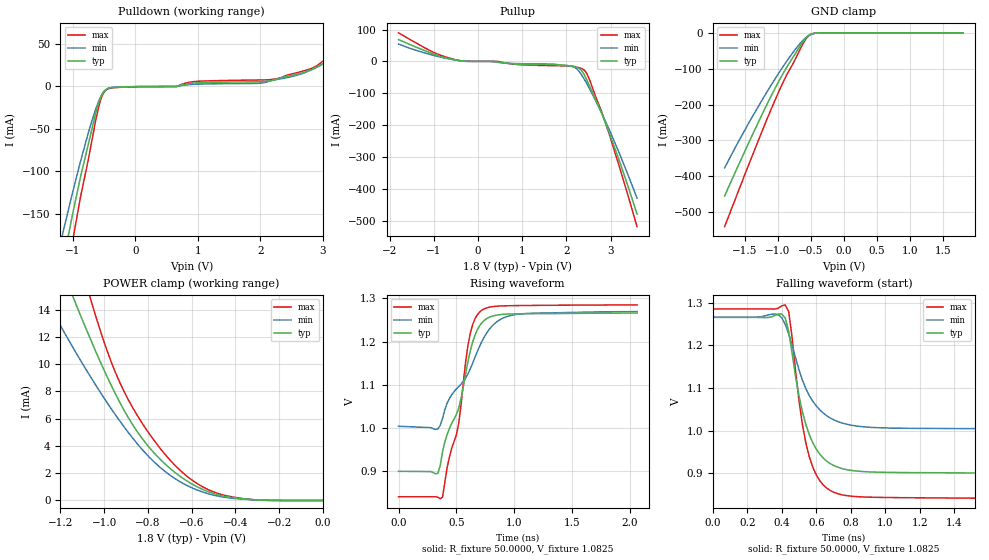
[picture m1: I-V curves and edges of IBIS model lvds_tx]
| Texas Instruments Incorporated
| 10bit, w200-MSPS, 4-channel/ 12bit, 80-MSPS, 8-Channel ADC
| Marketing part#   Voltage Range   Package-type   #pins/pkg drawing
| ADS5296   1.7V - 1.9V   QFN   64/QFN
[IBIS ver] 4.1
[File name] ads5296.ibs
[File Rev] 1.0
[Date] Mon Nov 16 17:09:14 IST 2009
[Source]   TIspice3 simulations
   Texas Instruments Incorporated.
   Analog eLab Design Center, HPA
   12500 TI Blvd
   Dallas, TX -75243
   For Support e-mail: elab_scm_ibis@list.ti.com
[Disclaimer]  Please be aware that in the absence of a written agreement,
   Texas Instruments (TI) assumes no liability for: 1)
   the accuracy of the IBIS models provided to your company, 2)
   the proper functioning of these IBIS models in your design or
   for any resulting applications, or; 3) infringement of patents,
   copyrights, or intellectual property rights resulting from
   your use of these IBIS models. TI provides IBIS models as a
   service to our customers and therefore reserves the right to
   limit distribution of the IBIS models.
[Copyright] (C)Copyright 2013 Texas Instruments Incorporated.
   All rights reserved.
|   Component ADS529xIPFP
[Component] ADS529xIPFP
[Manufacturer] Texas Instruments.
[Package]
| variable   typ   min   max
R_pkg   0.3702   0.1484   0.5035
L_pkg   3.6148nH   2.8818nH   4.60713nH
C_pkg   0.6034pF   0.5489pF   0.7199pF
[Pin]  signal_name   model_name   R_pin   L_pin   C_pin
1   TERM   TERM   NA   NA   NA
2   TERM   TERM   NA   NA   NA
3   TERM   TERM   NA   NA   NA
4   TERM   TERM   NA   NA   NA
5   TERM   TERM   NA   NA   NA
6   AGND   GND   NA   NA   NA
7   TERM   TERM   NA   NA   NA
8   TERM   TERM   NA   NA   NA
9   AGND   GND   NA   NA   NA
10   TERM   TERM   NA   NA   NA
11   TERM   TERM   NA   NA   NA
12   LGND   GND   NA   NA   NA
13   TERM   TERM   NA   NA   NA
14   LGND   GND   NA   NA   NA
15   OUT0_P   lvds_tx   NA   NA   NA
16   OUT0_N   lvds_tx   NA   NA   NA
17   OUT1_P   lvds_tx   NA   NA   NA
18   OUT1_N   lvds_tx   NA   NA   NA
19   OUT2_P   lvds_tx   NA   NA   NA
20   OUT2_N   lvds_tx   NA   NA   NA
21   OUT3_P   lvds_tx   NA   NA   NA
22   OUT3_N   lvds_tx   NA   NA   NA
23   ADCLKP   lvds_tx   NA   NA   NA
24   ADCLKN   lvds_tx   NA   NA   NA
25   LCLKP   lvds_tx   NA   NA   NA
26   LCLKN   lvds_tx   NA   NA   NA
27   OUT4_P   lvds_tx   NA   NA   NA
28   OUT4_N   lvds_tx   NA   NA   NA
29   OUT5_P   lvds_tx   NA   NA   NA
30   OUT5_N   lvds_tx   NA   NA   NA
31   OUT6_P   lvds_tx   NA   NA   NA
32   OUT6_N   lvds_tx   NA   NA   NA
33   OUT7_P   lvds_tx   NA   NA   NA
34   OUT7_N   lvds_tx   NA   NA   NA
35   LVDD   POWER   NA   NA   NA
36   LGND   GND   NA   NA   NA
37   AGND   GND   NA   NA   NA
38   TERM   TERM   NA   NA   NA
39   TERM   TERM   NA   NA   NA
40   AGND   GND   NA   NA   NA
41   TERM   TERM   NA   NA   NA
42   TERM   TERM   NA   NA   NA
43   AGND   GND   NA   NA   NA
44   TERM   TERM   NA   NA   NA
45   TERM   TERM   NA   NA   NA
46   AGND   GND   NA   NA   NA
47   TERM   TERM   NA   NA   NA
48   TERM   TERM   NA   NA   NA
49   TERM   TERM   NA   NA   NA
50   AVDD   POWER   NA   NA   NA
51   NC   NC   NA   NA   NA
52   TERM   TERM   NA   NA   NA
53   TERM   TERM   NA   NA   NA
54   TERM   TERM   NA   NA   NA
55   TERM   TERM   NA   NA   NA
56   TERM   TERM   NA   NA   NA
57   AVDD   POWER   NA   NA   NA
58   TERM   TERM   NA   NA   NA
59   TERM   TERM   NA   NA   NA
60   AVDD   POWER   NA   NA   NA
61   TERM   TERM   NA   NA   NA
62   TERM   TERM   NA   NA   NA
63   TERM   TERM   NA   NA   NA
64   TERM   TERM   NA   NA   NA
[Diff Pin]   inv_pin   vdiff   tdelay_typ   tdelay_min   tdelay_max
   15   16   350mV   0   0   0
   17   18   350mV   0   0   0
   19   20   350mV   0   0   0
   21   22   350mV   0   0   0
   23   24   350mV   0   0   0
   25   26   350mV   0   0   0
   27   28   350mV   0   0   0
   29   30   350mV   0   0   0
   31   32   350mV   0   0   0
   33   34   350mV   0   0   0
[Model]  TERM
Model_type Terminator
C_comp   0   0   0
[Voltage Range]  1.80  1.7  1.9
[Temperature Range] 25   125   -40
| Models and submodels in the file (2): lvds_tx (3-state), TERM (Terminator)
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|   Model lvds_tx
[Model]  lvds_tx
Model_type 3-state
Polarity   Non-Inverting
Enable   Active-Low
Vmeas = 1.065V
Cref = 5.0000pF
Rref = 50.0000
Vref = 1.065V
C_comp   2.2000pF   2.0000pF   2.4000pF
[Temperature Range]   25.0000   0.1250k   -40.0000
[Voltage Range]   1.8000V   1.7000V   1.9000V
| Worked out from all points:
|   slope of the pulldown table from 0 to 0.27 V, typ, clamps not added: 2.11 kohm
|   slope of the pullup table from 0 to 0.27 V, typ, clamps not added: 19.6 kohm
|   GND clamp passes 1 mA (typ) near -0.43 V on its own axis
|   POWER clamp passes 1 mA (typ) near -0.57 V on its own axis
|   rising waveform, R_fixture 50.0000, V_fixture 1.0825: 20-80 % time 228ps typ, 334ps min, 166ps max; typ from 0.899 V to 1.27 V
|   falling waveform, R_fixture 50.0000, V_fixture 1.0825: 20-80 % time 123ps typ, 153ps min, 102ps max; typ from 1.27 V to 0.899 V
[Pulldown]
|Voltage   I(typ)   I(min)   I(max)
-1.8V     -470.2mA   -385.4mA   -558.6mA
-1.19V    -219.2mA   -181mA     -264.4mA
-1.01V    -151.8mA   -126mA     -183.9mA
-880mV    -106.9mA   -88.53mA   -130.3mA
-640mV    -32.81mA   -27.64mA   -41.41mA
-550mV    -11.73mA   -11.48mA   -14.39mA
-450mV    -2.729mA   -2.929mA   -3.419mA
1.96V     5.415mA    3.576mA    7.487mA
2.3V      9.5mA      8.509mA    9.592mA
2.9V      22.47mA    22.43mA    24.06mA
3.29V     40.54mA    39.73mA    44.96mA
3.6V      59.26mA    55.48mA    67.55mA
[Pullup]
|Voltage   I(typ)   I(min)   I(max)
-1.8V     68.69mA    54.82mA    90mA
-990mV    22.5mA     18.4mA     27.38mA
-430mV    2.65mA     3.069mA    2.778mA
2.07V     -14.19mA   -13.88mA   -14.08mA
2.23V     -18.57mA   -22.67mA   -17.47mA
2.33V     -26.46mA   -39.19mA   -21.49mA
2.4V      -40.27mA   -54.59mA   -26.6mA
2.47V     -60.22mA   -71.58mA   -39.92mA
2.53V     -78.99mA   -86.98mA   -59.14mA
2.8V      -163.4mA   -162.4mA   -158.2mA
3.2V      -312.1mA   -288.5mA   -330.8mA
3.6V      -479.7mA   -429.6mA   -518.9mA
[GND_clamp]
|Voltage   I(typ)   I(min)   I(max)
-1.8V     -455.1mA   -376.5mA   -540.2mA
-1.43V    -303.7mA   -249.2mA   -364.1mA
-1.22V    -221.5mA   -182.7mA   -267.1mA
-1.03V    -151.6mA   -125.8mA   -183.6mA
-890mV    -104.4mA   -86.38mA   -127.2mA
-720mV    -54.06mA   -42.92mA   -68.61mA
-610mV    -22.22mA   -19.42mA   -27.81mA
-570mV    -13.4mA    -12.7mA    -16.38mA
-530mV    -7.078mA   -7.493mA   -8.285mA
-460mV    -1.728mA   -2.279mA   -1.919mA
-350mV    -129.4uA   -208.1uA   -178uA
1.8V      2.877nA    325.1nA    670.9pA
[POWER_clamp]
|Voltage   I(typ)   I(min)   I(max)
-1.8V     43.85mA    37.19mA    59.49mA
-1.26V    19.83mA    14.59mA    26.34mA
-1.13V    14.44mA    10.87mA    18.54mA
-1.09V    12.87mA    9.791mA    16.28mA
-1.04V    10.98mA    8.496mA    13.59mA
-950mV    7.865mA    6.317mA    9.449mA
-870mV    5.564mA    4.585mA    6.82mA
-770mV    3.457mA    2.802mA    4.368mA
-620mV    1.416mA    1.09mA     1.761mA
-520mV    624.2uA    477.4uA    765.1uA
-410mV    215.3uA    156.5uA    252.9uA
0V        2.877nA    37.47nA    895.7pA
[Ramp]
| variable   typ   min   max
dV/dt_r  0.7131/0.1616n   0.6999/0.2518n   0.7178/0.1193n
dV/dt_f  0.4975/0.2548n   0.4545/0.4195n   0.5349/0.1799n
R_load = 1.0000k
[Rising Waveform]
R_fixture= 50.0000
V_fixture= 1.0825
V_fixture_min= 1.1350
V_fixture_max= 1.0630
|time   V(typ)   V(min)   V(max)
0s        899mV      1.004V     840mV
340ps     894.4mV    997.3mV    838.9mV
380ps     943.7mV    1.022V     839mV
420ps     984.4mV    1.057V     908mV
520ps     1.045V     1.096V     1.01V
580ps     1.126V     1.115V     1.154V
620ps     1.178V     1.137V     1.219V
720ps     1.244V     1.2V       1.273V
980ps     1.264V     1.261V     1.283V
2.06ns    1.266V     1.269V     1.285V
[Falling Waveform]
R_fixture= 50.0000
V_fixture= 1.0825
V_fixture_min= 1.1350
V_fixture_max= 1.0630
|time   V(typ)   V(min)   V(max)
0s        1.266V     1.267V     1.286V
360ps     1.271V     1.274V     1.286V
420ps     1.265V     1.25V      1.295V
440ps     1.234V     1.227V     1.28V
500ps     1.081V     1.143V     1.07V
560ps     989.8mV    1.082V     937.9mV
620ps     944.7mV    1.049V     882.4mV
700ps     918.2mV    1.026V     855.3mV
980ps     902.1mV    1.007V     842.9mV
2.44ns    899.4mV    1.004V     840mV
